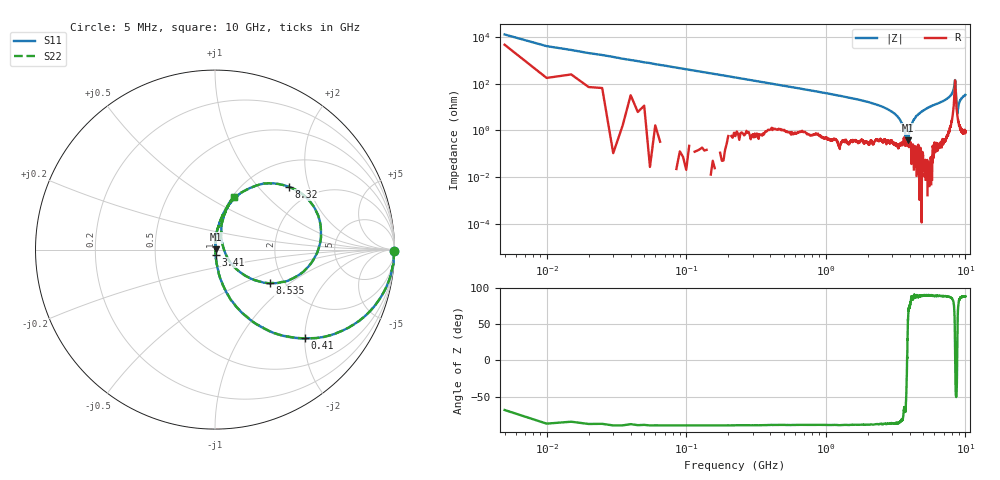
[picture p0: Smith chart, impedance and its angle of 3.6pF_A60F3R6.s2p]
! Amotech Co.,Ltd.
! http://www.amotech.co.kr/
! Part Number: A60F3R6
! These Parameters are Measured in Series Mode Connection
! Operation Temp=25[degC], DC Bias Voltage=0[V]
! Freq. Start=5[MHz] Stop=10[GHz], 2000[Steps]
! Date: Monday, July 20, 2020, 04:01:51
# GHZ S RI R 50.000000
!Freq.(Hz) S11(Real) S11(Imag) S21(Real) S21(Imag) S12(Real) S12(Imag) S22(Real) S22(Imag)
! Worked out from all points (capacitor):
!   2000 points, 5 MHz to 10 GHz, reference 50 ohm
!   read as one part in series: C = 3.85 pF near 55 MHz
!   lowest |Z| = 377 mohm at 3.855 GHz (marker M1)
!   series resonance near 3.822 GHz, so ESL is about 450 pH
!   S11 on the Smith chart (normalised r, x): 5 MHz: open; 410 MHz: 1.03, -1.99; 3.41 GHz: 1.01, -0.06; 8.32 GHz: 1.52, +1.50; 8.535 GHz: 1.68, -0.72; 10 GHz: 1.02, +0.66
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0.005  0.9971 -0.00731  0.00292 0.00731  0.00292 0.00731  0.9971 -0.00731
0.065  0.9754 -0.1545  0.0246 0.1545  0.0246 0.1545  0.9754 -0.1545
0.115  0.929 -0.2567  0.071 0.2567  0.071 0.2567  0.929 -0.2567
0.41  0.4987 -0.4935  0.5013 0.4935  0.5013 0.4935  0.4987 -0.4935
0.87  0.1753 -0.373  0.8247 0.373  0.8247 0.373  0.1753 -0.373
1.675  0.0463 -0.2022  0.9537 0.2022  0.9537 0.2022  0.0463 -0.2022
2.76  0.0098 -0.0813  0.9902 0.0813  0.9902 0.0813  0.0098 -0.0813
3.34  0.00363 -0.033  0.9964 0.033  0.9964 0.033  0.00363 -0.033
3.41  0.00356 -0.0278  0.9964 0.0278  0.9964 0.0278  0.00356 -0.0278
3.855  0.00318 0.002  0.9968 -0.002  0.9968 -0.002  0.00318 0.002
4.045  0.00285 0.0147  0.9971 -0.0147  0.9971 -0.0147  0.00285 0.0147
4.245  0.00237 0.0278  0.9976 -0.0278  0.9976 -0.0278  0.00237 0.0278
5.005  0.00541 0.0721  0.9946 -0.0721  0.9946 -0.0721  0.00541 0.0721
6.67  0.0286 0.1572  0.9714 -0.1572  0.9714 -0.1572  0.0286 0.1572
7.91  0.1124 0.2882  0.8876 -0.2882  0.8876 -0.2882  0.1124 0.2882
8.32  0.4139 0.3489  0.5861 -0.3489  0.5861 -0.3489  0.4139 0.3489
8.335  0.4473 0.3352  0.5527 -0.3352  0.5527 -0.3352  0.4473 0.3352
8.435  0.588 0.0476  0.412 -0.0476  0.412 -0.0476  0.588 0.0476
8.535  0.3038 -0.1878  0.6962 0.1878  0.6962 0.1878  0.3038 -0.1878
8.755  0.0447 0.0198  0.9553 -0.0198  0.9553 -0.0198  0.0447 0.0198
9.135  0.0452 0.1716  0.9548 -0.1716  0.9548 -0.1716  0.0452 0.1716
10  0.1045 0.2928  0.8955 -0.2928  0.8955 -0.2928  0.1045 0.2928
